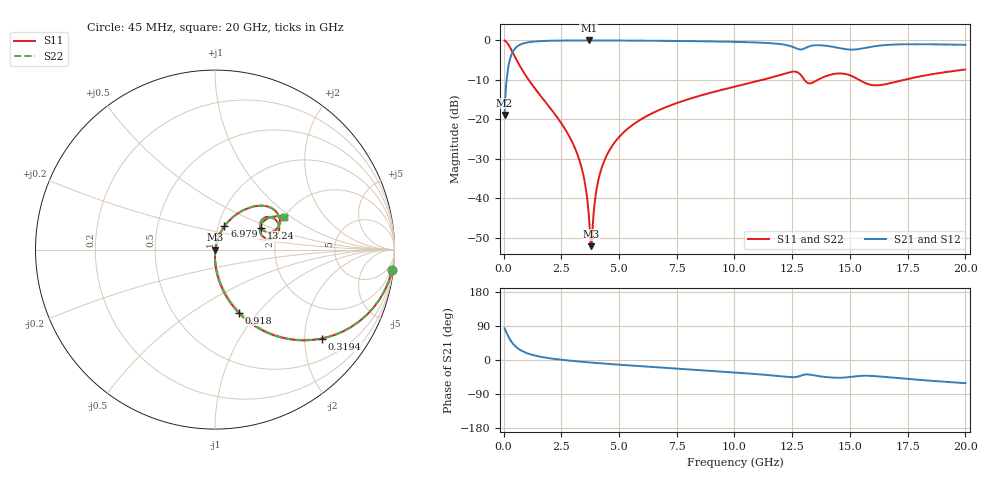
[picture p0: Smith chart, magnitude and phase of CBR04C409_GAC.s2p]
! S-parameter model data by Modelithics Inc.  support@modelithics.com 813-866-6335  Tampa FL USA
! S-Parameter data specifications:
! Substrate: 20-mil Rogers 4350B, substrate thickness, H=0.508mm, Dielectric constant, Er=3.75
! PCB Mounting Pad Footprint: Pad width, PadW=0.52mm , Pad length, PadL=0.52mm , Pad gap, PadG (edge-to-edge)=0.28mm , Reference planes=1.32mm apart
#  GHz  S  MA  R 50
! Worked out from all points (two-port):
!   801 points, 45 MHz to 20 GHz, reference 50 ohm
!   highest |S21| = -0.02 dB at 3.687 GHz (marker M1); lowest = -18.9 dB at 45 MHz (marker M2)
!   |S21| within 3 dB of the highest: 390.3 MHz to end of sweep
!   lowest |S11| = -52.1 dB at 3.787 GHz (marker M3), VSWR 1.00, Z = 50.2 - j0.0576 ohm
!   |S11| at or under -10 dB: 1.087 GHz to 11.2 GHz (10.12 GHz wide, 165 % of centre); 13.03 GHz to 13.6 GHz (576.6 MHz wide, 4.33 % of centre); 15.4 GHz to 17.33 GHz (1.931 GHz wide, 11.8 % of centre)
!   |S22| runs from -52.1 to -0.1 dB; largest |S21 - S12| = 0
!   S11 on the Smith chart (normalised r, x): 45 MHz: 1, -17; 319.4 MHz: 0.98, -2.43; 918 MHz: 0.98, -0.80; 6.979 GHz: 1.07, +0.29; 13.24 GHz: 1.62, +0.43; 20 GHz: 1.99, +0.89
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0.045  0.9936 -6.6  0.1132 83.4  0.1132 83.4  0.9936 -6.6
0.194662  0.8964 -26.6  0.443 63.3  0.443 63.3  0.8964 -26.6
0.319381  0.7751 -39.7  0.6313 50.2  0.6313 50.2  0.7751 -39.7
0.593762  0.544 -58.0  0.8382 31.9  0.8382 31.9  0.544 -58.0
0.918031  0.3752 -69.4  0.9257 20.4  0.9257 20.4  0.3752 -69.4
2.689037  0.07321 -89.0  0.9952 -0.6  0.9952 -0.6  0.07321 -89.0
3.387462  0.02386 -89.1  0.9973 -4.7  0.9973 -4.7  0.02386 -89.1
3.562069  0.01337 -85.3  0.9974 -5.6  0.9974 -5.6  0.01337 -85.3
3.686787  0.006392 -73.9  0.9974 -6.3  0.9974 -6.3  0.006392 -73.9
3.786563  0.002482 -13.4  0.9974 -6.8  0.9974 -6.8  0.002482 -13.4
4.110831  0.01729 73.1  0.9971 -8.3  0.9971 -8.3  0.01729 73.1
4.559819  0.03943 75.6  0.9964 -10.4  0.9964 -10.4  0.03943 75.6
5.382962  0.07639 73.7  0.9939 -14.0  0.9939 -14.0  0.07639 73.7
6.704981  0.13 69.0  0.9877 -19.5  0.9877 -19.5  0.13 69.0
6.979362  0.1407 67.9  0.9861 -20.6  0.9861 -20.6  0.1407 67.9
10.0225  0.2602 55.3  0.9576 -33.0  0.9576 -33.0  0.2602 55.3
12.54182  0.4022 30.6  0.8229 -45.4  0.8229 -45.4  0.4022 30.6
13.24024  0.285 25.3  0.8401 -38.5  0.8401 -38.5  0.285 25.3
13.36496  0.2904 29.5  0.8583 -39.6  0.8583 -39.6  0.2904 29.5
14.58721  0.3813 21.6  0.7944 -46.8  0.7944 -46.8  0.3813 21.6
16.68248  0.2846 27.3  0.8782 -45.6  0.8782 -45.6  0.2846 27.3
20  0.4277 25.4  0.8779 -61.1  0.8779 -61.1  0.4277 25.4
